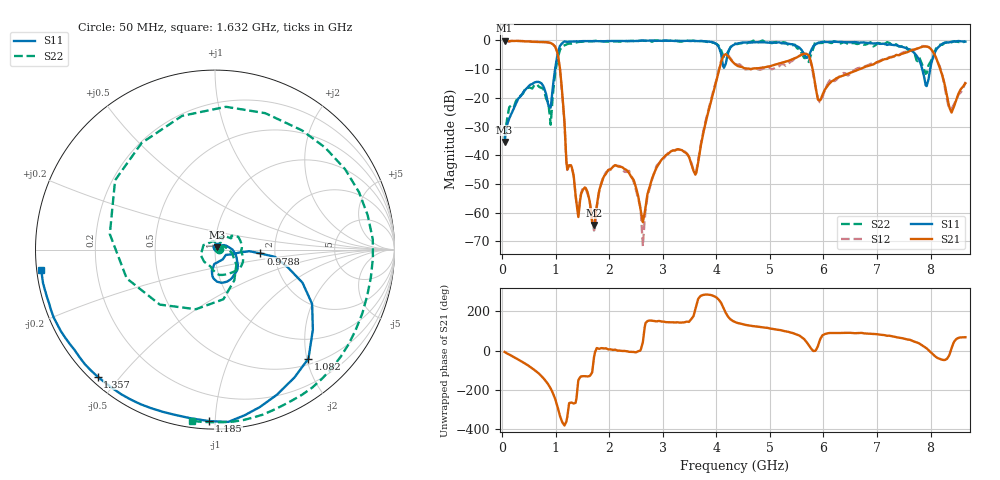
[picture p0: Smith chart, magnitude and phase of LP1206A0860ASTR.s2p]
!Instrument: 	"HEWLETT PACKARD,8720ES,US39172150,7.62 "
!	AVX THIN FILM OPERATION
!	LP1206 High Performance Low Pass Filters
!	P/N LP1206A0860ASTR  9 September 2018
!Instrument: 	"HEWLETT PACKARD,8720ES,US39172150,7.62 "
# MHz S dB R 50
!  Frq	S11(dB)	S11(deg)	S21(dB)	S21(deg)	S12(dB)	S12(deg)	S22(dB)	S22(deg)
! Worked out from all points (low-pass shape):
!   501 points, 50 MHz to 8.65 GHz, reference 50 ohm
!   highest |S21| = -0.06 dB at 50 MHz (marker M1); lowest = -64.2 dB at 1.718 GHz (marker M2)
!   |S21| within 3 dB of the highest: start of sweep to 1.013 GHz; 7.712 GHz to 8.009 GHz (297.5 MHz wide, 3.79 % of centre)
!   lowest |S11| = -35.3 dB at 50 MHz (marker M3), VSWR 1.03, Z = 51.1 + j1.32 ohm
!   |S11| at or under -10 dB: start of sweep to 992.1 MHz; 7.845 GHz to 7.993 GHz (147.8 MHz wide, 1.87 % of centre)
!   |S22| runs from -34.1 to 0.0 dB; largest |S21 - S12| = 0.065
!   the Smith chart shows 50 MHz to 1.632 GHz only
!   S11 on the Smith chart (normalised r, x): 50 MHz: 1.02, +0.03; 978.8 MHz: 1.68, -0.08; 1.082 GHz: 0.60, -2.03; 1.185 GHz: 0.04, -0.97; 1.357 GHz: 0.02, -0.44; 1.632 GHz: 0.01, -0.06
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50  -35.30 48.6  -0.06 -7.1  -0.09 -7.3  -34.13 2.3
617.6  -14.56 -62.3  -0.45 -101.0  -0.52 -101.2  -15.39 -23.6
858.4  -21.92 -92.7  -0.66 -169.5  -0.71 -169.9  -21.42 -158.7
978.8  -11.89 -4.8  -1.86 124.7  -1.91 124.4  -13.89 -57.8
1082  -1.94 -49.4  -9.54 29.2  -9.84 25.1  -3.38 145.2
1185.2  -0.39 -91.9  -35.31 -10.5  -35.70 -6.0  -1.55 42.8
1357.2  -0.32 -132.7  -50.51 92.7  -50.60 93.8  -0.80 -35.1
1494.8  -0.24 -154.7  -52.73 -130.6  -52.21 -133.3  -0.43 -70.4
1632.4  -0.23 -173.2  -55.51 -129.9  -55.52 -128.9  -0.33 -97.5
1718.4  -0.23 176.6  -64.22 -34.7  -66.20 -50.3  -0.20 -111.2
2148.4  -0.19 133.8  -43.74 0.6  -43.55 -1.4  -0.29 -168.6
2630  -0.02 92.2  -63.28 41.8  -71.63 62.5  -0.04 143.0
2922.4  -0.08 70.5  -43.17 150.2  -42.89 149.3  0.00 118.0
3610.4  -0.16 18.3  -46.71 -149.7  -46.12 -144.7  -0.30 61.9
4109.2  -6.79 -38.9  -6.56 -128.7  -6.23 -132.0  -4.33 10.3
4350  -1.30 -9.3  -8.22 144.8  -8.24 142.8  -1.09 19.7
5794.8  -2.60 -94.3  -9.68 2.5  -10.34 4.5  -3.54 -54.4
6224.8  -0.45 -141.8  -13.40 89.1  -13.92 92.6  -0.44 -108.6
7222.4  -1.39 142.5  -6.07 75.3  -5.90 74.9  -0.78 167.4
7927.6  -15.89 126.7  -2.13 11.0  -2.14 8.7  -11.35 171.6
8374.8  -0.54 108.1  -24.40 -2.7  -23.84 6.3  -0.64 123.3
8650  -0.39 82.7  -14.91 67.7  -14.41 72.9  -0.33 97.0
